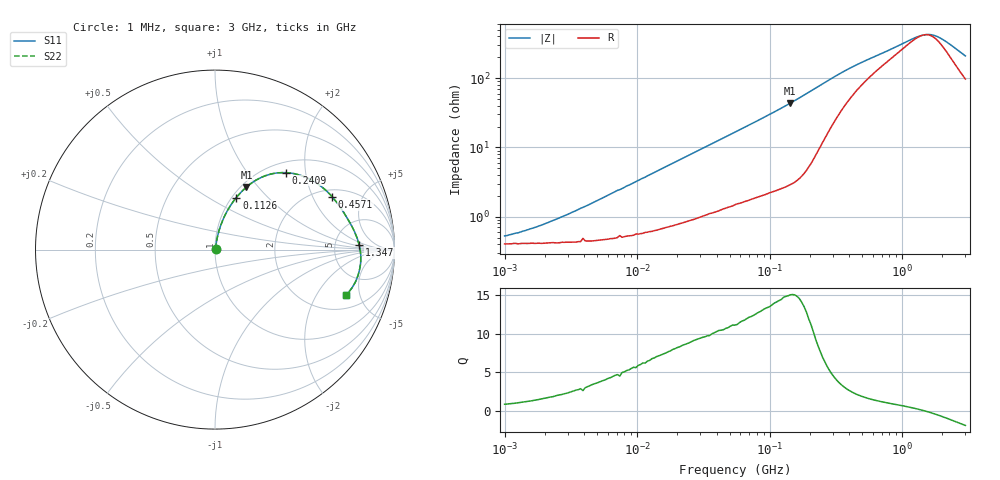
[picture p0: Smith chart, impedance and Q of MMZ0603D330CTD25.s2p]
! S-parameter Generated by TDK Corporation
! Copyright(C) 2018 TDK Corporation.
! All Rights Reserved.
! TDK P/N: MMZ0603D330CTD25 (Chip Bead)
! Property: |Z|=33¶ at 100MHz
! Size(LxWxT): 0.6x0.3x0.3mm, 0.024x0.012x0.012inches
! Model Type: s2p (Touchstone File Format Version 1.0)
! Frequency: DC=Yes Start=1MHz Stop=3000MHz 202points Log-sweep
! Model Generated on Aug. 6, 2018
! Port Assignments:
!  1 ---@@@--- 2
! Applicable Conditions:
!  Temperature = 25 degC
!  DC Bias Current = 0 A
!  Small Signal Operation
! Terms and conditions regarding TDK Simulation Models
! (1)This simulation model is being provided solely for informational purposes. Please refer to the specifications of the products in terms of detailed characteristics of such products.
! (2)In no event shall TDK Corporation of any of its subsidiaries be liable for any loss or damage arising, directly or indirectly,
!  From any information contained in this simulation model, including, but not limited to loss or damages arising from any inaccuracies, omissions or errors in connection with such information.
! (3)Any and all copyrights on this simulation model are owned by TDK Corporation.
!  Duplication or redistribution of this simulation model without prior written permission from TDK Corporation is prohibited.
! (4)This simulation model is subject to any modification or change without any prior notice.
! (5)Neither TDK Corporation nor any of its subsidiaries shall make any warranty, express or implied,
!  Including but not limited to the correctness, implied warranties of merchantability and fitness for a particular purpose with respect to this simulation models.
! (6)The use of this simulation model shall be deemed to have consented to the terms and conditions hereof.
# Hz S MA R 50
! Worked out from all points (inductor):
!   201 points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, 1 MHz to 3 GHz, reference 50 ohm
!   read as one part in series: L = 52.4 nH near 4.226 MHz
!   highest Q = 15 at 143.2 MHz (marker M1), where L = 48.3 nH
!   self-resonance near 1.467 GHz
!   S11 on the Smith chart (normalised r, x): 1 MHz: 1.01, +0.01; 112.6 MHz: 1.05, +0.67; 240.9 MHz: 1.20, +1.57; 457.1 MHz: 2.35, +2.84; 1.347 GHz: 8.98, +1.34; 3 GHz: 2.94, -3.71
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1000000  0.00527 39.9  0.996 -0.2  0.996 -0.2  0.00527 39.9
1271492  0.005846 46.1  0.996 -0.2  0.996 -0.2  0.005846 46.1
1897447  0.007515 56.6  0.9959 -0.4  0.9959 -0.4  0.007515 56.6
3900413  0.01356 68.3  0.9951 -0.7  0.9951 -0.7  0.01356 68.3
1.461624e7  0.04673 79.4  0.9924 -2.7  0.9924 -2.7  0.04673 79.4
3.00453e7  0.0923 78.7  0.986 -5.3  0.986 -5.3  0.0923 78.7
5.477226e7  0.1616 75.6  0.9725 -9.3  0.9725 -9.3  0.1616 75.6
8.173662e7  0.2339 72.0  0.9541 -13.5  0.9541 -13.5  0.2339 72.0
1.125904e8  0.3136 67.7  0.9276 -18.2  0.9276 -18.2  0.3136 67.7
1.431579e8  0.39 63.3  0.8953 -22.9  0.8953 -22.9  0.39 63.3
1.748812e8  0.4645 58.3  0.8532 -27.6  0.8532 -27.6  0.4645 58.3
2.136344e8  0.542 51.8  0.7893 -32.6  0.7893 -32.6  0.542 51.8
2.408952e8  0.5845 47.2  0.7396 -35.4  0.7396 -35.4  0.5845 47.2
2.827291e8  0.6324 40.8  0.665 -38.4  0.665 -38.4  0.6324 40.8
3.318279e8  0.6695 34.6  0.5882 -40.3  0.5882 -40.3  0.6695 34.6
4.570858e8  0.7158 24.3  0.4553 -40.3  0.4553 -40.3  0.7158 24.3
8.005644e8  0.7631 12.0  0.2989 -32.0  0.2989 -32.0  0.7631 12.0
1.347129e9  0.8036 1.9  0.1986 -7.7  0.1986 -7.7  0.8036 1.9
1.581072e9  0.8119 -1.7  0.19 7.4  0.19 7.4  0.8119 -1.7
1.855641e9  0.8148 -5.7  0.2056 23.1  0.2056 23.1  0.8148 -5.7
2.359433e9  0.8054 -12.1  0.2718 38.5  0.2718 38.5  0.8054 -12.1
3e9  0.7734 -19.1  0.3697 43.2  0.3697 43.2  0.7734 -19.1
